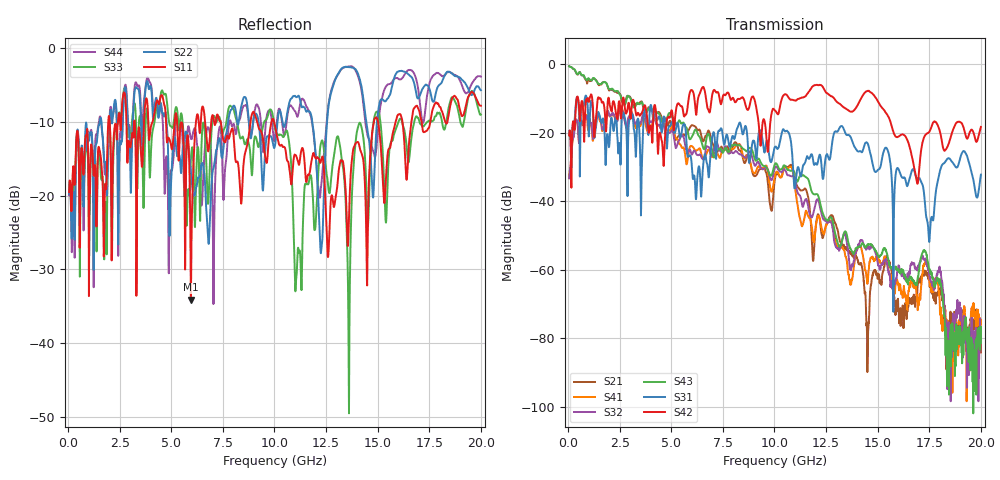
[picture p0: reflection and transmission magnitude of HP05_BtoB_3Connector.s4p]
# MHz S MA R 50.00
! FREQ  S11  S12  S13  S14
!  S21  S22  S23  S24
!  S31  S32  S33  S34
!  S41  S42  S43  S44
!  MAG  ANG  MAG  ANG  MAG  ANG  MAG  ANG
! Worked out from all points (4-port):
!   1996 points, 50 MHz to 20 GHz, reference 50 ohm
!   strongest paths, dB at 50 MHz, 5.04 GHz, 10.03 GHz, 15.02 GHz, 20 GHz:
!     S42: -20.8, -13.8, -13.5, -10.9, -18.3
!     S31: -20.8, -16.8, -24.1, -30.8, -32.2
!     S43: -0.6, -15.5, -29.0, -55.9, -78.7
!     S32: -33.3, -19.3, -30.1, -58.6, -79.2
!     S41: -33.3, -18.1, -32.4, -56.9, -78.6
!     S21: -0.5, -18.1, -33.2, -61.7, -84.2
!   lowest |S11| = -34.1 dB at 5.95 GHz (marker M1), VSWR 1.04, Z = 48.3 + j0.987 ohm
!   |S11| at or under -10 dB: start of sweep to 1.947 GHz; 7.398 GHz to 8.832 GHz (1.434 GHz wide, 17.7 % of centre); 9.98 GHz to 14.81 GHz (4.833 GHz wide, 39 % of centre)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
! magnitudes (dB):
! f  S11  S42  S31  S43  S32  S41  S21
! 50 MHz  -19.5  -20.8  -20.8  -0.6  -33.3  -33.3  -0.5
! 5.95 GHz  -34.1  -7.6  -27.1  -21.6  -25.7  -23.8  -18.0
! 12.26 GHz  -15.2  -6.1  -28.3  -41.8  -43.2  -47.2  -48.8
! 13.6 GHz  -23.8  -13.6  -20.7  -52.6  -56.2  -61.4  -54.7
! 14.1 GHz  -13.1  -11.1  -25.4  -53.3  -52.4  -53.2  -58.4
! 16.9 GHz  -7.8  -34.4  -33.5  -64.1  -60.0  -67.7  -67.4
! 20 GHz  -7.8  -18.3  -32.2  -78.7  -79.2  -78.6  -84.2
